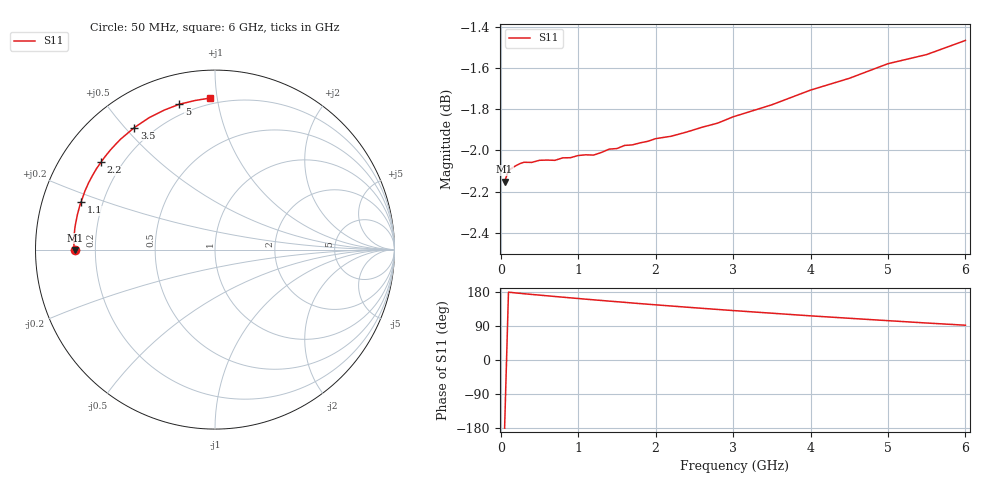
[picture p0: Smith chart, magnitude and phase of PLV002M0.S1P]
! Infineon Technologies  Discrete & RF Semiconductors
! BAR 64-04W /-05W /-06W
! Si PIN Diode in SOT323
! IF = 2 mA
! S-Parameters:  October  2008
# GHz  S  MA  R  50
!  f  S11
! GHz  MAG  ANG
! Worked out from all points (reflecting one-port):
!   34 points, 50 MHz to 6 GHz, reference 50 ohm
!   lowest |S11| = -2.2 dB at 50 MHz (marker M1), VSWR 8.11, Z = 6.16 - j0.0859 ohm
!   phase of S11 starts at -180 deg and turns -88 deg over the sweep
!   S11 on the Smith chart (normalised r, x): 50 MHz: 0.12, -0.00; 1.1 GHz: 0.12, +0.17; 2.2 GHz: 0.12, +0.33; 3.5 GHz: 0.13, +0.53; 5 GHz: 0.15, +0.77; 6 GHz: 0.16, +0.96
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0.05  0.7805 -179.8
0.1  0.7854 179.0
0.2  0.7876 176.8
0.25  0.7885 175.9
0.3  0.7891 174.9
0.4  0.789 173.0
0.5  0.79 171.2
0.8  0.791 165.8
0.9  0.7911 164.0
1  0.7921 162.3
1.1  0.7924 160.5
1.2  0.7923 158.8
1.4  0.7949 155.4
1.6  0.7965 152.2
1.7  0.7968 150.4
1.8  0.7977 148.8
2  0.7996 145.6
2.2  0.8006 142.5
2.4  0.8025 139.4
2.6  0.8047 136.4
2.8  0.8065 133.4
3  0.8094 130.5
3.5  0.8149 123.5
4  0.8216 116.5
4.5  0.827 110.1
5  0.8338 103.8
5.5  0.8381 97.6
6  0.8447 91.8
